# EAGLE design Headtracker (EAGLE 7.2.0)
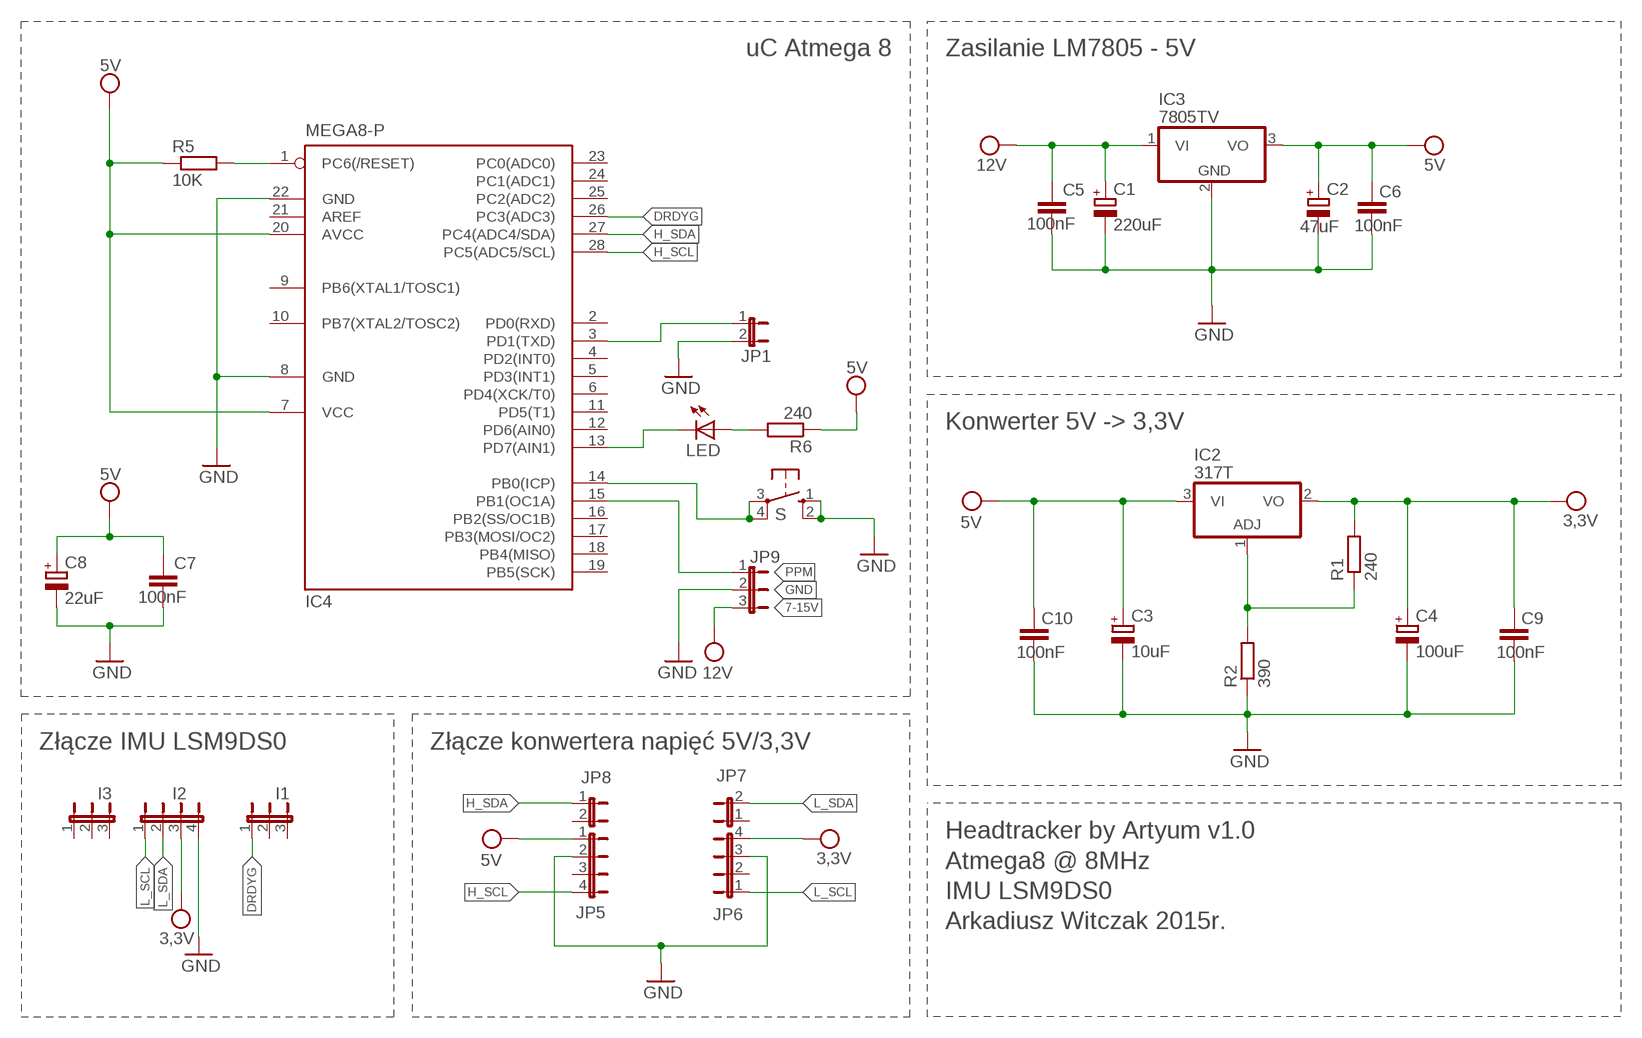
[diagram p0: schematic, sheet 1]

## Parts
C1  220uF  CPOL-EUE2.5-6  [E2,5-6]
C2  47uF  CPOL-EUE2.5-6  [E2,5-6]
C3  10uF  CPOL-EUE2.5-5  [E2,5-5]
C4  100uF  CPOL-EUE2.5-5  [E2,5-5]
C5  100nF  C-EU025-030X050  [C025-030X050]
C6  100nF  C-EU025-030X050  [C025-030X050]
C7  100nF  C-EU025-030X050  [C025-030X050]
C8  22uF  CPOL-EUE2.5-5  [E2,5-5]
C9  100nF  C-EU025-030X050  [C025-030X050]
C10  100nF  C-EU025-030X050  [C025-030X050]
I1  JP2E  [JP2]
I2  JP4E  [JP4]
I3  JP2E  [JP2]
IC2  317T  [TO220H]
IC3  7805TV  [TO220V]
IC4  MEGA8-P  [DIL28-3]
JP1  JP1E  [JP1]
JP5  JP4E  [JP4]
JP6  JP4E  [JP4]
JP7  JP1E  [JP1]
JP8  JP1E  [JP1]
JP9  JP2E  [JP2]
LED  LED5MM  [LED5MM]
R1  240  R-EU_0204/7  [0204/7]
R2  390  R-EU_0207/7  [0207/7]
R5  10K  R-EU_0204/7  [0204/7]
R6  240  R-EU_0204/7  [0204/7]
S  10-XX  [B3F-10XX]

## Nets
3,3V: C4.+ C9.1 I2.3 IC2.2(VO) JP6.4 R1.2
5V: C2.+ C3.+ C6.1 C7.1 C8.+ C10.1 IC2.3(VI) IC3.3(VO) IC4.7(VCC) IC4.20(AVCC) JP5.1 R5.1 R6.1
7-15V: JP9.3 ; supply symbol labelled 12V
12V: C1.+ C5.1 IC3.1(VI)
DRDYG: I1.1 IC4.26(PC3(ADC3))
GND: C1.- C2.- C3.- C4.- C5.2 C6.2 C7.2 C8.- C9.2 C10.2 I2.4 IC3.2(GND) IC4.8(GND) IC4.22(GND) JP1.2 JP5.2 JP6.3 JP9.2 R2.1 S.1(S) S.2(S1)
H_SCL: IC4.28(PC5(ADC5/SCL)) JP5.4
H_SDA: IC4.27(PC4(ADC4/SDA)) JP8.1
L_SCL: I2.1 JP6.1
L_SDA: I2.2 JP7.2
N$3: IC4.13(PD7(AIN1)) LED.K(C)
N$4: LED.A R6.2
N$6: IC2.1(ADJ) R1.1 R2.2
N$7: IC4.14(PB0(ICP)) S.3(P) S.4(P1)
PPM: IC4.15(PB1(OC1A)) JP9.1
RST: IC4.1(PC6(/RESET)) R5.2
TX: IC4.3(PD1(TXD)) JP1.1
Unconnected: I1.2 I1.3 I3.1 I3.2 I3.3 IC4.2(PD0(RXD)) IC4.4(PD2(INT0)) IC4.5(PD3(INT1)) IC4.6(PD4(XCK/T0)) IC4.9(PB6(XTAL1/TOSC1)) IC4.10(PB7(XTAL2/TOSC2)) IC4.11(PD5(T1)) IC4.12(PD6(AIN0)) IC4.16(PB2(SS/OC1B)) IC4.17(PB3(MOSI/OC2)) IC4.18(PB4(MISO)) IC4.19(PB5(SCK)) IC4.21(AREF) IC4.23(PC0(ADC0)) IC4.24(PC1(ADC1)) IC4.25(PC2(ADC2)) JP5.3 JP6.2 JP7.1 JP8.2

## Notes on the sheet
- uC Atmega 8
- Zasilanie LM7805 - 5V
- Konwerter 5V -> 3,3V
- Złącze IMU LSM9DS0 | Złącze konwertera napięć 5V/3,3V
- Headtracker by Artyum v1.0
  Atmega8 @ 8MHz
  IMU LSM9DS0
  Arkadiusz Witczak 2015r.

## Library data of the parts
C1-C4 C8 = rcl:CPOL-EU: POLARIZED CAPACITOR, European symbol
C5-C7 C9 C10 = rcl:C-EU: CAPACITOR, European symbol
I1 I3 JP9 = jumper:JP2E: JUMPER
I2 JP5 JP6 = jumper:JP4E: JUMPER
IC2 = linear:*317: Positive VOLTAGE REGULATOR
IC3 = linear:78*: Positive VOLTAGE REGULATOR Source: http://cache.national.com/ds/LM/LM78L05.pdf http://www.fairchildsemi.com/ds/LM/LM7805.pdf
IC4 = atmel:MEGA8-P: MICROCONTROLLER 8 Kbytes FLASH, 1 kbytes SRAM, 512 bytes EEPROM, USART, 4-channel 10 bit ADC, 2-channel 8 bit ADC Pin compatible with Atmega48, ATMega88, ATMega168 Source: avr.lbr; OC_FARNELL: unknown; OC_NEWARK: unknown
JP1 JP7 JP8 = jumper:JP1E: JUMPER
LED = led:LED: LED
R1 R2 R5 R6 = rcl:R-EU_: RESISTOR, European symbol
S = switch-omron:10-XX: OMRON SWITCH; MPN: B3F-1000; OC_FARNELL: 176432; OC_NEWARK: 36M3542

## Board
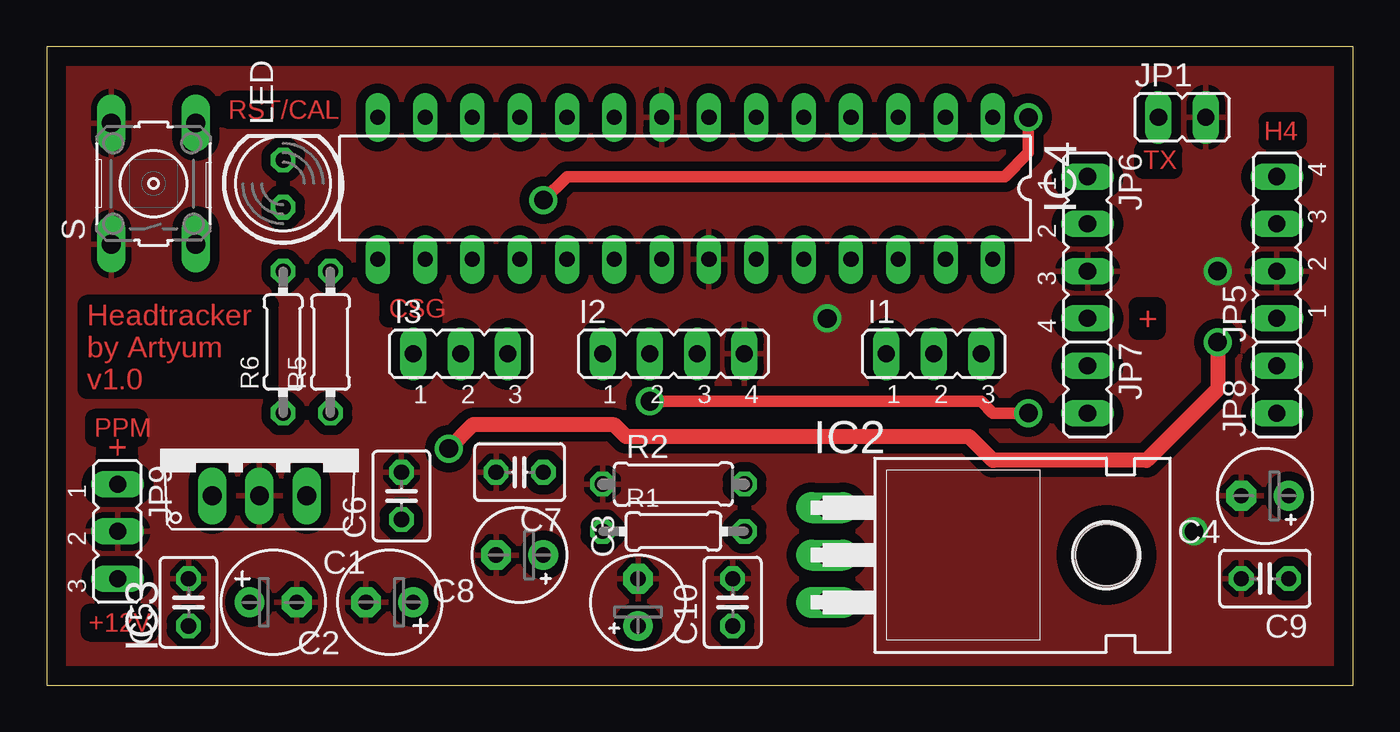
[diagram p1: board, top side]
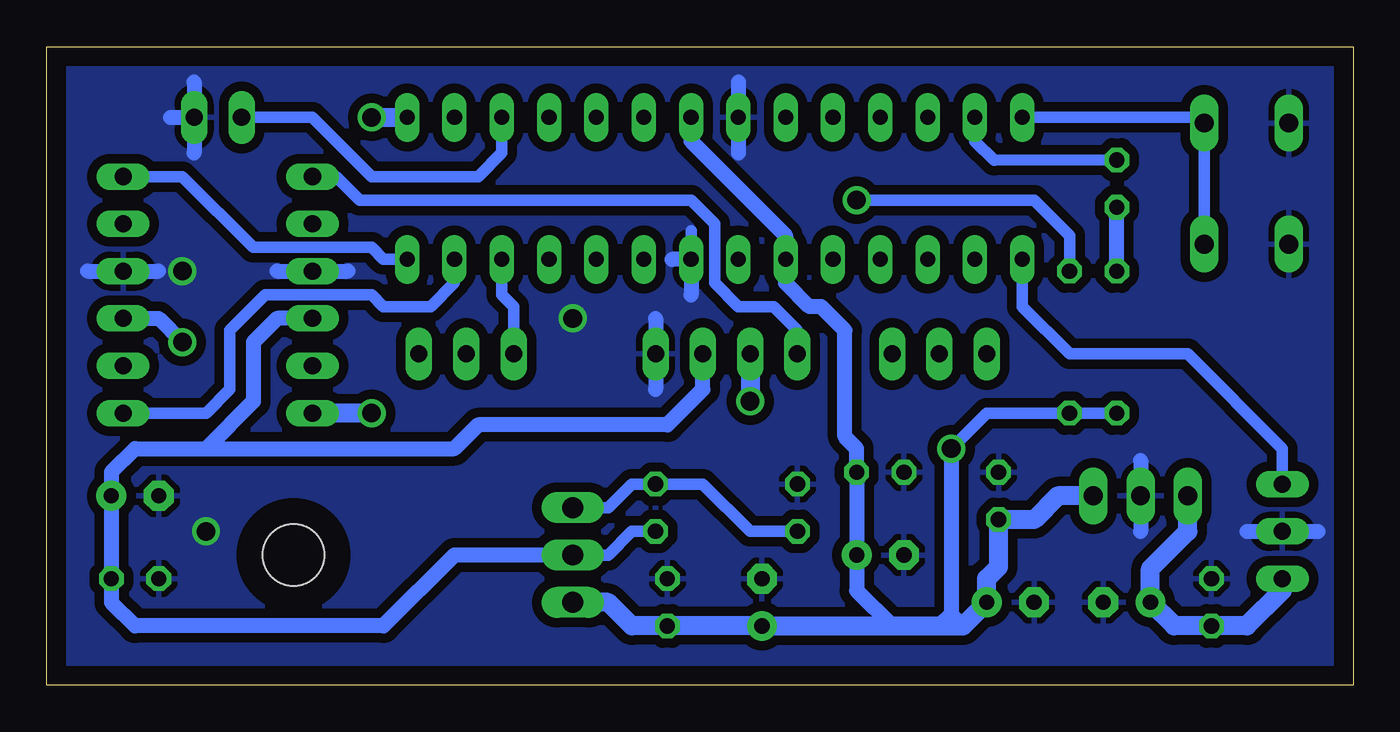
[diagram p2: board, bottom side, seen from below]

Size 70.16 x 34.28 mm. Coordinates in mm from the lower left corner, seen from the top.
Outline: 0,0 70.16,0 70.16,34.28 0,34.28 0,0
Copper layers (1*16): Top 0.035mm / dielectric 1.5mm / Bottom 0.035mm
Design rules "default *": minimum track width 10mil, minimum drill 24mil, track to track 8mil, track to pad 8mil, pad to pad 8mil, via to via 8mil, smd to smd 8mil, copper to edge 40mil, drill to drill 8mil, minimum pad ring 10mil, minimum via ring 8mil, stop-mask expansion 4mil, vias tented up to drill 0mil, thermal gap 13mil

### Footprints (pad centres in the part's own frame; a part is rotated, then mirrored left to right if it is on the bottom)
E2,5-6 = drill 0.813 pad 1.6: + -1.27,0 | drill 0.813 pad 1.6 octagon: - 1.27,0
E2,5-5 = drill 0.813 pad 1.6: + -1.27,0 | drill 0.813 pad 1.6 octagon: - 1.27,0
C025-030X050 = drill 0.813 octagon: 1 -1.27,0; 2 1.27,0
JP2 = drill 0.914 long: 1 -2.54,0; 2 0,0; 3 2.54,0
JP4 = drill 0.914 long: 1 -3.81,0; 2 -1.27,0; 3 1.27,0; 4 3.81,0
TO220H = drill 1.118 long: 1 -2.54,-10.16; 2 0,-10.16; 3 2.54,-10.16 | hole 3.302: 0,4.826
TO220V = drill 1.016 long: 1 -2.54,-2.54; 2 0,-2.54; 3 2.54,-2.54
DIL28-3 = drill 0.813 long: 1 -16.51,-3.81; 2 -13.97,-3.81; 3 -11.43,-3.81; 4 -8.89,-3.81; 5 -6.35,-3.81; 6 -3.81,-3.81; 7 -1.27,-3.81; 8 1.27,-3.81; 9 3.81,-3.81; 10 6.35,-3.81; 11 8.89,-3.81; 12 11.43,-3.81; 13 13.97,-3.81; 14 16.51,-3.81; 15 16.51,3.81; 16 13.97,3.81; 17 11.43,3.81; 18 8.89,3.81; 19 6.35,3.81; 20 3.81,3.81; 21 1.27,3.81; 22 -1.27,3.81; 23 -3.81,3.81; 24 -6.35,3.81; 25 -8.89,3.81; 26 -11.43,3.81; 27 -13.97,3.81; 28 -16.51,3.81
JP1 = drill 0.914 long: 1 0,-1.27; 2 0,1.27
LED5MM = drill 0.813 octagon: A -1.27,0; K 1.27,0
0204/7 = drill 0.813 octagon: 1 -3.81,0; 2 3.81,0
0207/7 = drill 0.813 octagon: 1 -3.81,0; 2 3.81,0
B3F-10XX = drill 1.016 long: 1 -3.251,2.261; 2 3.251,2.261; 3 -3.251,-2.261; 4 3.251,-2.261

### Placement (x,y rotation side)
C1  12.17,4.45 0 top
C2  18.41,4.45 180 top
C3  31.75,4.45 90 top
C4  65.41,10.16 180 top
C5  7.62,4.45 90 top
C6  19.05,10.16 90 top
C7  25.4,11.43 180 top
C8  25.4,6.99 180 top
C9  65.41,5.72 180 top
C10  36.83,4.45 90 top
I1  47.62,17.78 0 top
I2  33.65,17.78 0 top
I3  22.23,17.78 0 top
IC2  52.07,6.99 270 top
IC3  11.43,12.7 0 top
IC4  34.29,26.67 180 top
JP1  60.96,30.48 270 top
JP5  66.04,23.5 90 top
JP6  55.88,23.5 270 top
JP7  55.88,15.88 180 top
JP8  66.04,15.88 0 top
JP9  3.81,8.25 270 top
LED  12.7,26.92 90 top
R1  33.65,8.25 0 top
R2  33.65,10.8 0 top
R5  15.24,18.41 90 top
R6  12.7,18.41 90 top
S  5.74,26.92 90 top

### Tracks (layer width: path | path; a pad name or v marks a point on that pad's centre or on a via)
3,3V
  Bottom 0.61: IC2.2 40,6.99 38.73,8.25 R1.2
  Bottom 0.813: IC2.2 48.26,6.99 52.07,3.17 65.41,3.17 66.67,4.45 C9.1 C4.+ 66.67,11.43 65.41,12.7 61.59,12.7 | 61.59,12.7 48.26,12.7 46.99,13.97 36.83,13.97 34.92,15.88 I2.3 | JP6.4 57.78,19.69 59.05,18.41 59.05,15.24 61.59,12.7
5V  (via drill 1)
  Top 0.813: v62.87,18.41 62.87,15.88 59.05,12.07 50.8,12.07 49.53,13.34 31.11,13.34 30.48,13.97 22.86,13.97 v21.59,12.7
  Bottom 0.61: R6.1 R5.1 19.68,14.61 v21.59,12.7
  Bottom 0.813: v21.59,12.7 21.59,3.81 | 21.59,3.81 20.96,3.17 | 21.59,3.81 22.23,3.17 | JP5.1 64.14,19.69 v62.87,18.41 | IC4.7 35.56,29.21 30.48,24.13 IC4.20 30.48,21.59 29.21,20.32 28.57,20.32 27.3,19.05 27.3,13.34 26.67,12.7 C7.1 C8.+ 26.67,5.08 24.77,3.17
  Bottom 1.016: IC2.3 40,4.45 38.73,3.17 C10.1 C3.+ 24.77,3.17 22.23,3.17 20.96,3.17 C2.+ 19.68,5.72 19.05,6.35 C6.1 17.14,8.89 15.88,10.16 IC3.3
12V
  Bottom 1.016: 3.81,5.08 5.71,3.17 C5.1 9.63,3.17 C1.+ 10.9,6.25 8.89,8.25 IC3.1
DRDYG
  Bottom 0.61: I1.1 45.08,20.32 45.72,20.96 IC4.26
GND  (via drill 1)
  Bottom 0.61: 35.56,24.38 IC4.22
  Bottom 0.813: 57.78,22.23 53.97,22.23 | 11.43,12.07 11.43,8.25 | 33.02,32.38 33.02,28.57 | 35.56,20.96 IC4.22 36.58,22.86 | 37.46,19.69 37.46,15.88 | 67.95,22.23 64.14,22.23 | 5.71,8.25 1.9,8.25 | 62.23,32.38 JP1.2 | JP1.2 62.23,28.57 | 63.5,30.48 JP1.2
  other vias: 61.59,8.25 62.87,22.23 41.91,19.69
  pour Bottom (isolate 0.508): -0.64,34.29 -0.64,0 70.48,0 70.48,34.29
  pour Top (isolate 0.508): -0.64,34.29 -0.64,-0.64 71.76,-0.64 71.76,34.29
H_SCL
  Bottom 0.61: JP5.4 62.87,27.3 59.05,23.5 52.7,23.5 52.07,22.86 IC4.28
H_SDA
  Bottom 0.61: IC4.27 48.26,21.59 49.53,20.32 52.07,20.32 52.7,20.96 58.42,20.96 60.32,19.05 60.32,15.88 61.59,14.61 JP8.1
L_SCL
  Bottom 0.61: I2.1 29.84,19.05 31.11,20.32 33.02,20.32 34.29,21.59 34.29,24.77 35.56,26.04 53.34,26.04 54.61,27.3 JP6.1
L_SDA  (via drill 1)
  Top 0.61: v32.38,15.24 50.16,15.24 50.8,14.61 v52.7,14.61
  Bottom 1.016: v52.7,14.61 JP7.2 | I2.2 v32.38,15.24
N$3
  Bottom 0.61: IC4.13 20.32,29.21 19.28,28.17 LED.K
N$4
  Bottom 0.813: R6.2 LED.A
N$6
  Bottom 0.61: IC2.1 40,9.52 38.73,10.8 R2.2 34.92,10.8 32.38,8.25 R1.1
N$7
  Bottom 0.61: IC4.14 8.31,30.48 S.4 S.3
PPM
  Bottom 0.61: IC4.15 17.78,20.32 15.24,17.78 8.89,17.78 3.81,12.7 JP9.1
RST  (via drill 1)
  Top 0.61: v26.67,26.04 27.94,27.3 51.43,27.3 52.7,28.57 v52.7,30.48
  Bottom 0.61: R5.2 15.24,24.13 17.14,26.04 v26.67,26.04
  Bottom 1.016: v52.7,30.48 IC4.1
TX
  Bottom 0.61: IC4.3 45.72,28.57 46.99,27.3 52.7,27.3 55.88,30.48 JP1.1

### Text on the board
Top: RST/CAL | H4 | TX | Headtracker / by Artyum / v1.0 | CSG | + | PPM | + | +12V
